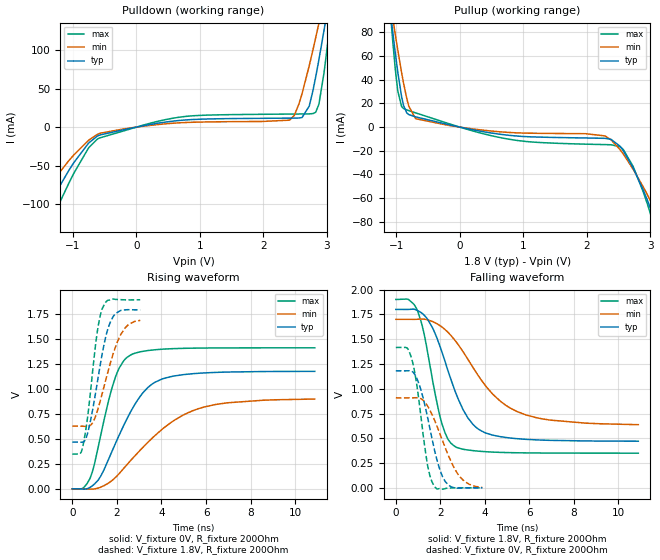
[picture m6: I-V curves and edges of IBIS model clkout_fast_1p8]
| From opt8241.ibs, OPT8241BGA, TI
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|   clkout_fast_1p8 Model
[Model]   clkout_fast_1p8
Model_type   Output
Polarity   Non-Inverting
Vmeas = 0.9
Vref = 0
Cref = 2pF
Rref = 200
|   typ   min   max
|   (nom PVT)   (fast PVT)   (slow PVT)
C_comp   2.233e-12   2.012e-12   2.445e-12
| Where nom  PVT is Nominal Process, 1.8V, 27C
|   Fast PVT is Strong Process,  1.9V, -40C
|   Slow PVT is Weak Process,   1.7V, 125C
[Voltage Range]   1.8   1.7   1.9
|Junction Temperature
[Temperature Range]   27   125   -40
[Pullup Reference]   1.8   1.7   1.9
[Pulldown Reference]   0   0   0
[Power Clamp Reference]   1.8   1.7   1.9
[GND Clamp Reference]   0   0   0
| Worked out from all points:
|   slope of the pulldown table from 0 to 0.27 V, typ, clamps not added: 65 ohm
|   slope of the pullup table from 0 to 0.27 V, typ, clamps not added: 93.1 ohm
|   falling waveform, V_fixture 1.8V, R_fixture 200Ohm: 20-80 % time 1.35ns typ, 2.19ns min, 825ps max; typ from 1.8 V to 0.471 V
|   rising waveform, V_fixture 0V, R_fixture 200Ohm: 20-80 % time 1.59ns typ, 2.62ns min, 924ps max; typ from 0 V to 1.18 V
|   rising waveform, V_fixture 1.8V, R_fixture 200Ohm: 20-80 % time 643ps typ, 828ps min, 480ps max; typ from 0.469 V to 1.8 V
|   falling waveform, V_fixture 0V, R_fixture 200Ohm: 20-80 % time 725ps typ, 1.01ns min, 513ps max; typ from 1.18 V to 0.001 V
[Pulldown]
|   Voltage   I(typ)   I(min)   I(max)
-1.8V     -258.1mA   -149.7mA   -365.8mA
-1.499V   -118mA     -89.3mA    -148.6mA
-981.1mV  -45.55mA   -35.7mA    -59.26mA
-574.2mV  -10.14mA   -7.949mA   -13.89mA
709.2mV   8.866mA    5.738mA    13.22mA
2.416V    11.65mA    9.106mA    16.92mA
2.608V    12.38mA    43.04mA    17.05mA
2.722V    27.14mA    79.32mA    17.18mA
2.822V    64.24mA    115.2mA    19.15mA
2.952V    123.8mA    163.6mA    68.75mA
3.077V    186.4mA    211.5mA    153.3mA
3.6V      457.2mA    410mA      548.9mA
[Pullup]
|   Voltage   I(typ)   I(min)   I(max)
-1.8V     458.1mA    373mA      626.4mA
-1.103V   101.4mA    108.4mA    102.2mA
-1.059V   80.92mA    92.67mA    73.34mA
-979.2mV  46.74mA    65.34mA    30.76mA
-918mV    25.62mA    45.98mA    17.35mA
-698.4mV  8.689mA    7.137mA    12.08mA
774.5mV   -6.9mA     -4.487mA   -10.22mA
2.287V    -9.463mA   -7.432mA   -14.76mA
2.574V    -20mA      -22.83mA   -19mA
2.952V    -61.68mA   -57.02mA   -64.89mA
3.323V    -114.5mA   -97.21mA   -129.2mA
3.6V      -250.6mA   -205.3mA   -271mA
[Ramp]
R_load = 200
|   typ   min   max
dV/dt_r   0.707996/1.58753e-09   0.543725/2.62913e-09   0.849334/9.23516e-10
dV/dt_f   0.798024/1.34746e-09   0.641287/2.20441e-09   0.929966/8.23377e-10
[Falling Waveform]
V_fixture = 1.8V
V_fixture_min = 1.7V
V_fixture_max = 1.9V
R_fixture = 200Ohm
|   Time   V(typ)   V(min)   V(max)
0s        1.8V       1.7V       1.9V
572ps     1.8V       1.7V       1.9V
982ps     1.788V     1.701V     1.782V
1.418ns   1.704V     1.695V     1.381V
2.048ns   1.387V     1.627V     667.8mV
2.358ns   1.174V     1.566V     486.8mV
2.72ns    943.9mV    1.471V     409.6mV
3.71ns    593.1mV    1.132V     370.5mV
5.432ns   496.6mV    772.1mV    354.3mV
10.91ns   470.8mV    637.4mV    350.2mV
[Rising Waveform]
V_fixture = 0V
V_fixture_min = 0V
V_fixture_max = 0V
R_fixture = 200Ohm
|   Time   V(typ)   V(min)   V(max)
0s        749.6pV    47.93nV    353.2pV
452ps     -1.461mV   226.7uV    3.786mV
798ps     15.03mV    -2.563mV   106.3mV
1.268ns   124.8mV    16.2mV     530.2mV
1.934ns   454.6mV    114mV      1.12V
2.298ns   632.9mV    203.9mV    1.283V
2.614ns   772.9mV    283.9mV    1.343V
3.702ns   1.069V     533.9mV    1.396V
5.702ns   1.161V     808mV      1.413V
10.87ns   1.179V     901.6mV    1.415V
[Rising Waveform]
V_fixture = 1.8V
V_fixture_min = 1.7V
V_fixture_max = 1.9V
R_fixture = 200Ohm
|   Time   V(typ)   V(min)   V(max)
0s        469.4mV    629.2mV    349.3mV
344ps     468.7mV    629.4mV    350.2mV
476ps     469.2mV    628.5mV    427.6mV
804ps     670.8mV    636.2mV    947.1mV
1.106ns   1.044V     769.2mV    1.553V
1.348ns   1.365V     961.6mV    1.811V
1.608ns   1.614V     1.182V     1.893V
1.884ns   1.745V     1.389V     1.904V
2.376ns   1.796V     1.617V     1.897V
3.046ns   1.796V     1.691V     1.898V
[Falling Waveform]
|Gnd
V_fixture = 0V
V_fixture_min = 0V
V_fixture_max = 0V
R_fixture = 200Ohm
|   Time   V(typ)   V(min)   V(max)
0s        1.181V     908.3mV    1.416V
500ps     1.181V     908.3mV    1.412V
706ps     1.178V     908.4mV    1.308V
1.032ns   1.055V     907mV      893.7mV
1.42ns    719.4mV    828.2mV    237.5mV
1.738ns   382.2mV    683.9mV    13.34mV
2.09ns    118.9mV    483.4mV    -12.86mV
2.38ns    26.45mV    318.5mV    -2.766mV
3.064ns   -1.141mV   70.04mV    1.312mV
3.892ns   1.36mV     5.559mV    291.1uV
